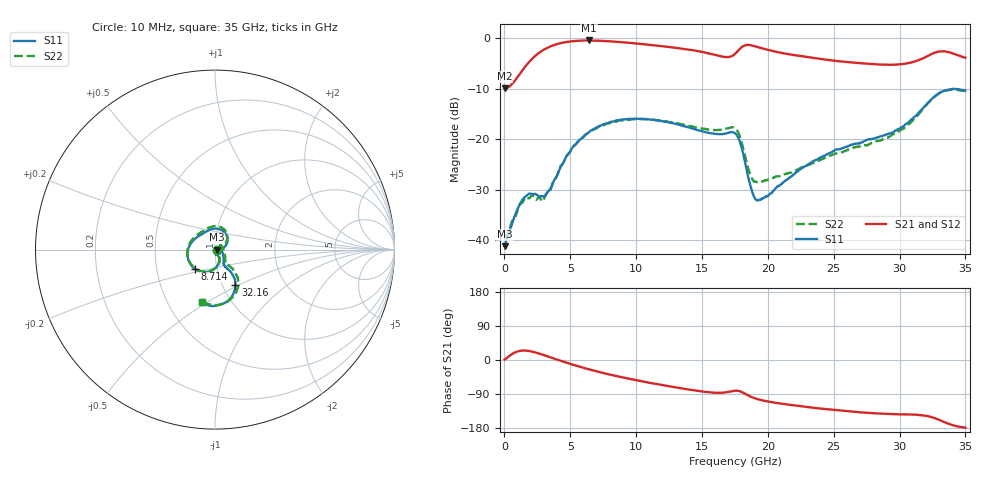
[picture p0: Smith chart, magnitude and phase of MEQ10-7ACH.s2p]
! MARKI MICROWAVE INC.
! Email:  support@markimicrowave.com  Phone:  408-778-4200
! Model Number:  MEQ10-7ACH  Date:  6/18
! Filename:		MEQ10-7ACH.S2P  Version: 1.0
! Description:  2-port S-parameter data for chip equalizer
! Features:		Low Insertion Loss, Excellent Return Loss
! Frequency Measured: 	10 MHz to 35 GHz
!S2P File: Measurements: S11, S21, S12, S22:
# Hz S  dB  R 50
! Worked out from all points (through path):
!   1601 points, 10 MHz to 35 GHz, reference 50 ohm
!   highest |S21| = -0.47 dB at 6.418 GHz (marker M1); lowest = -10.0 dB at 10 MHz (marker M2)
!   group delay of S21, straight-line fit = 15.2 ps
!   lowest |S11| = -41.2 dB at 10 MHz (marker M3), VSWR 1.02, Z = 50.9 - j0.0642 ohm
!   |S11| at or under -10 dB: start of sweep to end of sweep
!   |S22| runs from -39.3 to -10.2 dB; largest |S21 - S12| = 0.009
!   S11 on the Smith chart (normalised r, x): 10 MHz: 1.02, -0.00; 8.714 GHz: 0.78, -0.17; 32.16 GHz: 1.15, -0.48; 35 GHz: 0.73, -0.47
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1e7  -41.16 -4.1  -9.96 1.2  -9.86 1.7  -39.12 0.6
1.322125e9  -32.16 -44.5  -6.53 24.8  -6.53 24.8  -32.63 -38.5
2.393694e9  -30.89 -79.3  -3.38 19.4  -3.38 19.5  -31.97 -73.5
3.202838e9  -30.75 -71.6  -1.99 10.5  -1.99 10.4  -30.67 -62.0
4.449356e9  -24.73 -66.2  -0.89 -4.1  -0.89 -4.1  -24.78 -62.5
5.848956e9  -19.85 -88.7  -0.49 -19.1  -0.49 -19.1  -19.85 -86.7
6.417544e9  -18.61 -98.4  -0.47 -24.7  -0.46 -24.7  -18.74 -97.7
8.713762e9  -16.21 -135.4  -0.77 -43.9  -0.77 -44.0  -16.30 -136.7
1.168791e10  -16.32 -175.0  -1.53 -64.4  -1.51 -64.4  -16.23 -178.0
1.553681e10  -18.77 135.1  -3.04 -85.3  -3.03 -85.2  -18.11 130.9
1.687081e10  -18.82 104.4  -3.77 -85.0  -3.76 -85.2  -17.88 103.2
1.7505e10  -18.82 71.2  -3.12 -81.0  -3.13 -81.1  -17.83 73.7
1.789864e10  -20.66 41.1  -2.07 -82.8  -2.08 -82.9  -19.63 48.5
1.831414e10  -25.11 16.3  -1.41 -90.1  -1.42 -90.0  -23.81 31.5
1.877339e10  -30.07 12.5  -1.45 -97.9  -1.46 -97.7  -27.69 34.5
1.918889e10  -32.09 19.7  -1.74 -103.0  -1.72 -102.8  -28.45 41.4
2.334396e10  -24.53 -38.1  -3.88 -125.7  -3.88 -125.5  -24.75 -20.9
2.918291e10  -18.91 -59.4  -5.26 -142.5  -5.22 -142.6  -19.61 -50.6
3.101989e10  -15.85 -55.0  -4.74 -144.1  -4.77 -144.1  -16.22 -47.8
3.215706e10  -12.81 -60.3  -3.52 -148.2  -3.52 -147.8  -12.84 -54.9
3.344732e10  -10.36 -80.4  -2.63 -164.6  -2.57 -164.3  -10.42 -78.2
3.5e10  -10.38 -104.0  -3.89 -178.6  -3.79 -178.9  -10.45 -103.6
